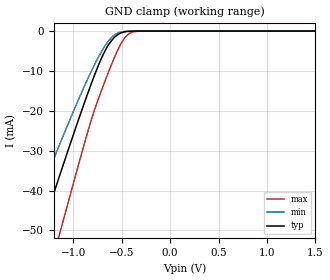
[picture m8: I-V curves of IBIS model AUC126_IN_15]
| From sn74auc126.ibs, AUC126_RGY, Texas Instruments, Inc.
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[Model]   AUC126_IN_15
Model_type  Input
Vinl=0.49
Vinh=1.04
| variable   typ   min   max
C_comp   2.35pF   1.94pF   2.69pF
[Temperature Range]   40   100   -40
| Ambient temperature   25   85   -40
[Voltage range]   1.5   1.4   1.6
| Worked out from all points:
|   GND clamp passes 1 mA (typ) near -0.55 V on its own axis
[GND Clamp]
| AUC126_IN_15
|   Voltage   I(typ)   I(min)   I(max)
-3.6V     -222.3mA   -186mA     -267.4mA
-1.505V   -63.39mA   -50.69mA   -83.42mA
-1.325V   -49.92mA   -39.59mA   -67.38mA
-1.17V    -38.45mA   -30.23mA   -53.54mA
-1.12V    -34.78mA   -27.27mA   -49.07mA
-840mV    -14.97mA   -11.47mA   -24.46mA
-695mV    -6.113mA   -4.618mA   -14.06mA
-570mV    -1.487mA   -910.9uA   -6.381mA
-495mV    -364.6uA   -178.7uA   -2.692mA
-430mV    -73.19uA   -34.72uA   -776.9uA
-280mV    -781.4nA   -556.2nA   -5.358uA
1.5V      165.9pA    258.5pA    172.1pA
